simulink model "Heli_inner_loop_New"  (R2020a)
settings: Solver=FixedStepDiscrete  StartTime=0.0  StopTime=10.0  FixedStep=0.01  RelTol=1e-3  EnableMultiTasking=on
model workspace (MAT data in the model file):
  Ts : Simulink.Parameter (value not decoded)
libraries: simulink x1

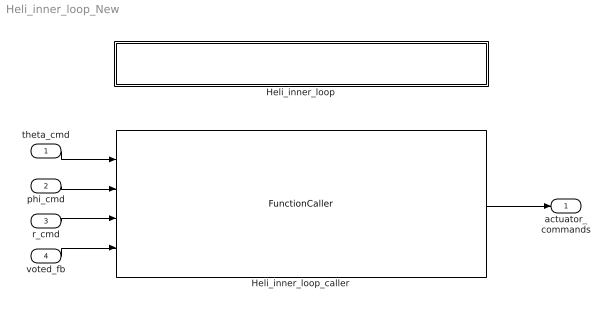
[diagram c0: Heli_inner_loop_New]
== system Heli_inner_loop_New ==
  theta_cmd : Inport
  phi_cmd : Inport  Port=2
  r_cmd : Inport  Port=3
  voted_fb : Inport  Port=4
  Heli_inner_loop : Subsystem  TreatAsAtomicUnit=on
  Heli_inner_loop_caller : FunctionCaller  FunctionPrototype=actuator_commands = Heli_inner_loop(theta_cmd,phi_cmd,r_cmd,voted_fb)
  actuator_commands : Outport
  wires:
  theta_cmd/1 -> Heli_inner_loop_caller/1
  phi_cmd/1 -> Heli_inner_loop_caller/2
  voted_fb/1 -> Heli_inner_loop_caller/4
  r_cmd/1 -> Heli_inner_loop_caller/3
  Heli_inner_loop_caller/1 -> actuator_commands/1

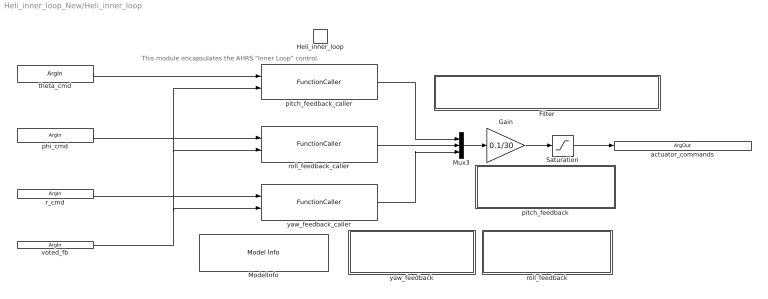
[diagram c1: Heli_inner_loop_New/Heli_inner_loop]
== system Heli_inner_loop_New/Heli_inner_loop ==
  note: This module encapsulates the AHRS "Inner Loop" control.
  Heli_inner_loop : TriggerPort  TriggerType=function-call  IsSimulinkFunction=on  FunctionName=Heli_inner_loop  FunctionVisibility=scoped  VariantControl=Variant  PortDimensions=1
  Filter : Subsystem  Tag=FilterWizardSubSystem  RequirementInfo={} %GIDa_ac7f675d_0c04_474f_b6aa_16ea1999b46b  TreatAsAtomicUnit=on  RTWFcnName=InnerLoopFilter
  Gain : Gain  Gain=0.1/30
  ModelInfo : simulink/Model-Wide Utilities/Model Info  Frame=on  DisplayStringWithTags=|  HorizontalTextAlignment=Center  LeftAlignmentValue=0.5
      | Model Name: %<ModelName>
      | Model Version: %<ModelVersion>
      | Last Modified: %<LastModificationDate>
      | 
      | Copyright 2016 The MathWorks, Inc.
  Mux3 : Mux  Inputs=3
  Saturation : Saturate  UpperLimit=0.1  LowerLimit=-0.1
  pitch_feedback : Subsystem  TreatAsAtomicUnit=on
  pitch_feedback_caller : FunctionCaller  FunctionPrototype=ds = pitch_feedback(theta_cmd,voted_fb)
  roll_feedback : Subsystem  TreatAsAtomicUnit=on
  roll_feedback_caller : FunctionCaller  FunctionPrototype=dc = roll_feedback(phi_cmd,voted_fb)
  yaw_feedback : Subsystem  TreatAsAtomicUnit=on
  yaw_feedback_caller : FunctionCaller  FunctionPrototype=dT = yaw_feedback(r_cmd,voted_fb)
  theta_cmd : ArgIn  ArgumentName=theta_cmd
  phi_cmd : ArgIn  Port=2  ArgumentName=phi_cmd
  r_cmd : ArgIn  Port=3  ArgumentName=r_cmd
  voted_fb : ArgIn  Port=4  PortDimensions=5  ArgumentName=voted_fb
  actuator_commands : ArgOut  PortDimensions=3  ArgumentName=actuator_commands
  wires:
  voted_fb/1 -> roll_feedback_caller/2, pitch_feedback_caller/2, yaw_feedback_caller/2
  Saturation/1 -> actuator_commands/1
  Gain/1 -> Saturation/1
  Mux3/1 -> Gain/1
  theta_cmd/1 -> pitch_feedback_caller/1
  phi_cmd/1 -> roll_feedback_caller/1
  r_cmd/1 -> yaw_feedback_caller/1
  roll_feedback_caller/1 -> Mux3/2
  yaw_feedback_caller/1 -> Mux3/3
  pitch_feedback_caller/1 -> Mux3/1

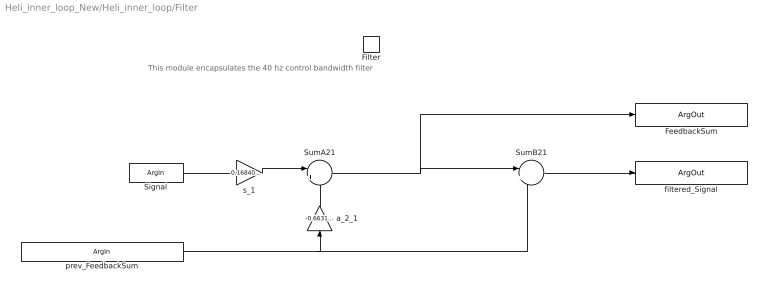
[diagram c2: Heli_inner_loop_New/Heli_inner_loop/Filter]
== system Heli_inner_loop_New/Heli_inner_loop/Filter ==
  note: This module encapsulates the 40 hz control bandwidth filter
  Filter : TriggerPort  TriggerType=function-call  IsSimulinkFunction=on  FunctionName=Filter  FunctionVisibility=scoped  VariantControl=Variant  PortDimensions=1
  SumA21 : Sum  Inputs=|+-  RndMeth=Zero  SaturateOnIntegerOverflow=on
  SumB21 : Sum  Inputs=|++  RndMeth=Zero  SaturateOnIntegerOverflow=on
  a_2_1 : Gain  Gain=-0.66319151740124993  ParamDataTypeStr=double  RndMeth=Zero  SaturateOnIntegerOverflow=on
  s_1 : Gain  Gain=0.16840424129937498  ParamDataTypeStr=double  RndMeth=Zero  SaturateOnIntegerOverflow=on
  Signal : ArgIn  ArgumentName=Signal
  prev_FeedbackSum : ArgIn  Port=2  ArgumentName=prev_FeedbackSum
  filtered_Signal : ArgOut  ArgumentName=filtered_Signal
  FeedbackSum : ArgOut  Port=2  ArgumentName=FeedbackSum
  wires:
  a_2_1/1 -> SumA21/2
  SumB21/1 -> filtered_Signal/1
  SumA21/1 -> FeedbackSum/1, SumB21/1
  s_1/1 -> SumA21/1
  Signal/1 -> s_1/1
  prev_FeedbackSum/1 -> SumB21/2, a_2_1/1

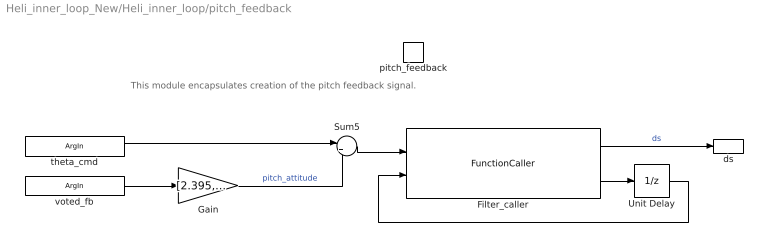
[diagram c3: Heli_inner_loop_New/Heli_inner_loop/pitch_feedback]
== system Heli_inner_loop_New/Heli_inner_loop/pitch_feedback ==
  note: This module encapsulates creation of the pitch feedback signal.
  pitch_feedback : TriggerPort  TriggerType=function-call  IsSimulinkFunction=on  FunctionName=pitch_feedback  FunctionVisibility=scoped  VariantControl=Variant  PortDimensions=1
  Filter_caller : FunctionCaller  FunctionPrototype=[filtered_Signal,FeedbackSum] = Filter(Signal,prev_FeedbackSum)  InputArgumentSpecifications=double(1), double(1)  OutputArgumentSpecifications=double(1), double(1)
  Gain : Gain  Gain=[2.395,-0.3609,-0.002145,0.8087,-0.0205;;;]  Multiplication=Matrix(K*u) (u vector)
  Sum5 : Sum  Inputs=|+-
  Unit Delay : UnitDelay  SampleTime=-1  HasFrameUpgradeWarning=on
  theta_cmd : ArgIn  ArgumentName=theta_cmd
  voted_fb : ArgIn  Port=2  PortDimensions=5  ArgumentName=voted_fb
  ds : ArgOut  ArgumentName=ds
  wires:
  voted_fb/1 -> Gain/1
  theta_cmd/1 -> Sum5/1
  Sum5/1 -> Filter_caller/1
  Filter_caller/1 -> ds/1  "ds"
  Gain/1 -> Sum5/2  "pitch_attitude"
  Filter_caller/2 -> Unit Delay/1
  Unit Delay/1 -> Filter_caller/2

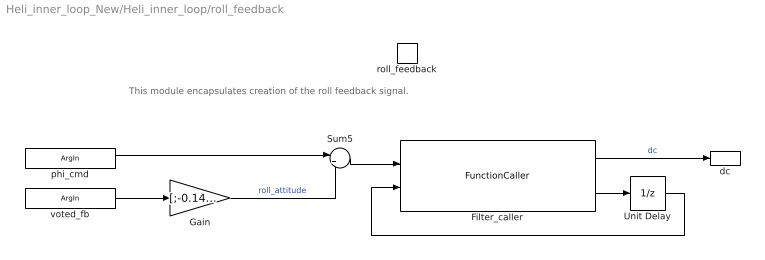
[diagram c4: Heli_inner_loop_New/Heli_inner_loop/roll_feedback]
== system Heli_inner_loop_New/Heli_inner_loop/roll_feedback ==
  note: This module encapsulates creation of the roll feedback signal.
  roll_feedback : TriggerPort  TriggerType=function-call  IsSimulinkFunction=on  FunctionName=roll_feedback  FunctionVisibility=scoped  VariantControl=Variant  PortDimensions=1
  Filter_caller : FunctionCaller  FunctionPrototype=[filtered_Signal,FeedbackSum] = Filter(Signal,prev_FeedbackSum)  InputArgumentSpecifications=double(1), double(1)  OutputArgumentSpecifications=double(1), double(1)
  Gain : Gain  Gain=[;-0.1427,-1.115,0.04573,-0.04318,-0.1007;;]  Multiplication=Matrix(K*u) (u vector)
  Sum5 : Sum  Inputs=|+-
  Unit Delay : UnitDelay  SampleTime=-1  HasFrameUpgradeWarning=on
  phi_cmd : ArgIn  ArgumentName=phi_cmd
  voted_fb : ArgIn  Port=2  PortDimensions=5  ArgumentName=voted_fb
  dc : ArgOut  ArgumentName=dc
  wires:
  Unit Delay/1 -> Filter_caller/2
  Filter_caller/2 -> Unit Delay/1
  Gain/1 -> Sum5/2  "roll_attitude"
  Filter_caller/1 -> dc/1  "dc"
  Sum5/1 -> Filter_caller/1
  phi_cmd/1 -> Sum5/1
  voted_fb/1 -> Gain/1

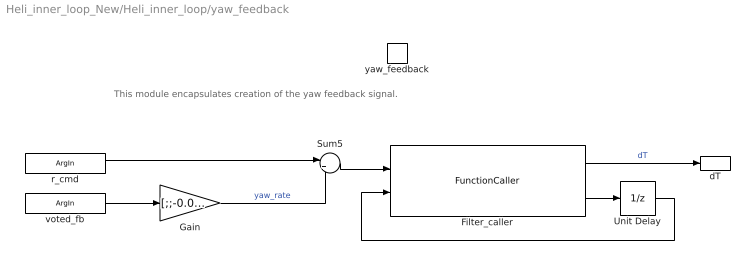
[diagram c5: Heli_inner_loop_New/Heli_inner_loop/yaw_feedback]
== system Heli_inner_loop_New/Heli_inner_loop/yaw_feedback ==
  note: This module encapsulates creation of the yaw feedback signal.
  yaw_feedback : TriggerPort  TriggerType=function-call  IsSimulinkFunction=on  FunctionName=yaw_feedback  FunctionVisibility=scoped  VariantControl=Variant  PortDimensions=1
  Filter_caller : FunctionCaller  FunctionPrototype=[filtered_Signal,FeedbackSum] = Filter(Signal,prev_FeedbackSum)  InputArgumentSpecifications=double(1), double(1)  OutputArgumentSpecifications=double(1), double(1)
  Gain : Gain  Gain=[;;-0.02792,-0.02229,-2.025,-0.06152,0.03151;]  Multiplication=Matrix(K*u) (u vector)
  Sum5 : Sum  Inputs=|+-
  Unit Delay : UnitDelay  SampleTime=-1  HasFrameUpgradeWarning=on
  r_cmd : ArgIn  ArgumentName=r_cmd
  voted_fb : ArgIn  Port=2  PortDimensions=5  ArgumentName=voted_fb
  dT : ArgOut  ArgumentName=dT
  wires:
  voted_fb/1 -> Gain/1
  r_cmd/1 -> Sum5/1
  Sum5/1 -> Filter_caller/1
  Filter_caller/1 -> dT/1  "dT"
  Gain/1 -> Sum5/2  "yaw_rate"
  Filter_caller/2 -> Unit Delay/1
  Unit Delay/1 -> Filter_caller/2
